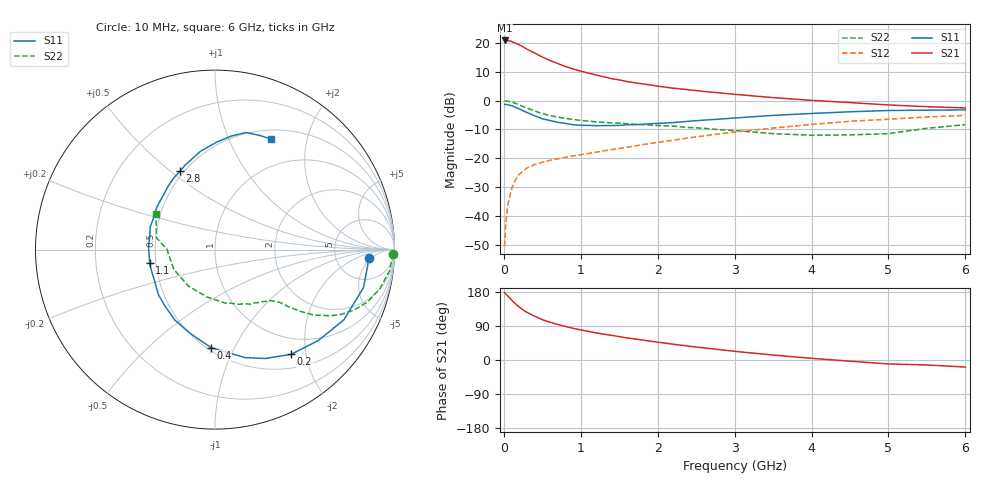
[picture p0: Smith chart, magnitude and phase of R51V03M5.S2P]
! SIEMENS Small Signal Semiconductors
! BFR183
! Si NPN RF Bipolar Junction Transistor in SOT23
! VCE = 1 V  IC = 3.5 mA
! Common Emitter S-Parameters:  May  1996
# GHz  S  MA  R  50
!  f  S11  S21  S12  S22
! GHz  MAG  ANG  MAG  ANG  MAG  ANG  MAG  ANG
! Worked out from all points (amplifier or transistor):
!   36 points, 10 MHz to 6 GHz, reference 50 ohm
!   highest |S21| = 20.9 dB at 10 MHz (marker M1)
!   |S21| within 3 dB of that: start of sweep to 300 MHz
!   unconditionally stable (mu >= 1): 1.137 GHz to 2.935 GHz
!   at 250 MHz: K = 0.34, MSG = 21.5 dB, |S12| = -24.4 dB
!   at 1.4 GHz: K = 1.07, MAG = 10.7 dB, |S12| = -17.0 dB
!   at 6 GHz: K = 0.94, MSG = 1.3 dB, |S12| = -5.1 dB
!   S11 on the Smith chart (normalised r, x): 10 MHz: 12, -4; 200 MHz: 0.71, -1.74; 400 MHz: 0.52, -0.81; 1.1 GHz: 0.46, -0.08; 2.8 GHz: 0.48, +0.54; 6 GHz: 0.61, +1.45
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0.01  0.8586 -3.0  11.05 178.1  0.003 85.5  0.991 -1.4
0.02  0.8553 -6.1  10.87 175.5  0.0061 81.8  0.9883 -2.7
0.05  0.8538 -14.4  10.96 169.1  0.0152 81.8  0.9796 -6.9
0.1  0.8177 -28.6  10.63 158.7  0.0295 75.6  0.9444 -13.3
0.15  0.7666 -41.4  9.893 148.5  0.0419 68.0  0.8991 -18.9
0.2  0.7211 -54.0  9.329 139.8  0.0527 63.3  0.8457 -23.4
0.25  0.6688 -65.1  8.579 132.1  0.0602 58.9  0.7902 -27.2
0.3  0.6246 -74.5  7.821 125.8  0.0678 56.1  0.7439 -29.7
0.4  0.5464 -92.4  6.683 115.5  0.0779 51.5  0.6619 -33.5
0.5  0.4855 -106.9  5.697 106.5  0.0852 49.1  0.5954 -35.6
0.6  0.4521 -119.6  4.967 99.7  0.0923 47.9  0.5502 -36.9
0.7  0.4209 -131.2  4.396 93.7  0.098 47.5  0.5192 -37.8
0.9  0.3821 -150.5  3.549 83.6  0.1101 47.9  0.471 -39.0
1.1  0.3725 -168.2  3.005 75.4  0.1214 49.2  0.4406 -40.9
1.3  0.3704 178.2  2.584 68.2  0.1347 50.2  0.4192 -42.7
1.6  0.3827 160.7  2.145 58.4  0.1557 51.1  0.3977 -46.7
2.2  0.4164 134.1  1.644 41.7  0.2064 51.0  0.3613 -57.2
2.8  0.4781 114.2  1.364 27.5  0.2656 47.6  0.3138 -72.6
3.5  0.5552 98.1  1.128 13.1  0.335 40.6  0.2676 -99.9
4.5  0.6405 81.6  0.925 -3.1  0.4386 28.1  0.2546 -154.0
5.5  0.6834 68.5  0.785 -13.1  0.5201 15.5  0.3316 168.7
6  0.691 63.0  0.748 -18.6  0.555 7.2  0.3834 149.2
